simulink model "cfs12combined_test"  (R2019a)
settings: configuration reference "configurationSettings" (kept in a data dictionary, not in this file)
undefined symbols (not defined in the file or in its folder): algo_cfs1_fp, algo_cfs2_fp

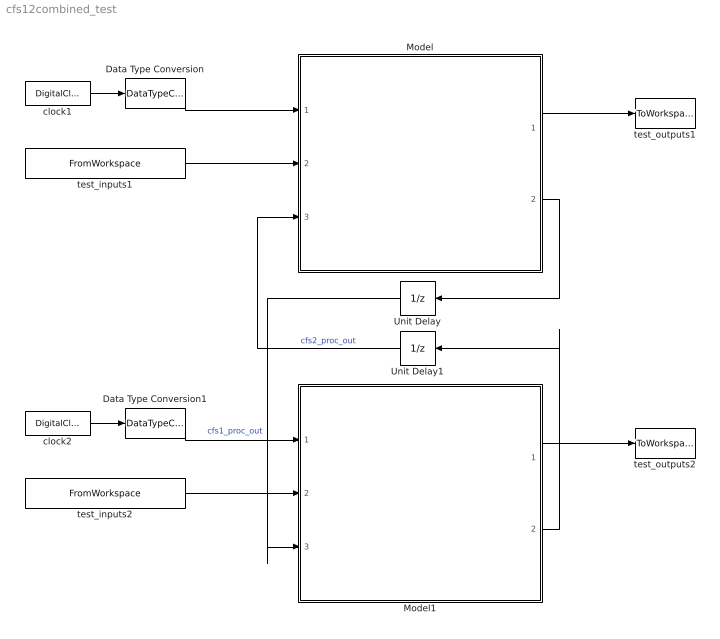
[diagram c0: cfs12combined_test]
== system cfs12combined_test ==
  Data Type Conversion : DataTypeConversion  OutDataTypeStr=single
  Data Type Conversion1 : DataTypeConversion  OutDataTypeStr=single
  Model : ModelReference  ModelNameDialog=algo_cfs1.slx  SimulationMode=Normal  ModelReferenceVersion=1.801  SimulationMode=Normal
  Model1 : ModelReference  ModelNameDialog=algo_cfs2.slx  SimulationMode=Normal  ModelReferenceVersion=1.795  SimulationMode=Normal
  Unit Delay : UnitDelay  SampleTime=-1  HasFrameUpgradeWarning=on
  Unit Delay1 : UnitDelay  SampleTime=-1  HasFrameUpgradeWarning=on
  clock1 : DigitalClock  SampleTime=algo_cfs1_fp.timing.dt
  clock2 : DigitalClock  SampleTime=algo_cfs1_fp.timing.dt
  test_inputs1 : FromWorkspace  VariableName=algo_cfs1_inbus1  OutDataTypeStr=Bus: algo_cfs1_inBus  SampleTime=algo_cfs1_fp.timing.dt  Interpolate=off  OutputAfterFinalValue=Holding final value
  test_inputs2 : FromWorkspace  VariableName=algo_cfs2_inbus1  OutDataTypeStr=Bus: algo_cfs2_inBus  SampleTime=algo_cfs2_fp.timing.dt  Interpolate=off  OutputAfterFinalValue=Holding final value
  test_outputs1 : ToWorkspace  VariableName=simout1  SaveFormat=Timeseries  SampleTime=-1
  test_outputs2 : ToWorkspace  VariableName=simout2  SaveFormat=Timeseries  SampleTime=-1
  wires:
  Model1/2 -> Unit Delay1/1
  clock2/1 -> Data Type Conversion1/1
  Unit Delay1/1 -> Model/3  "cfs2_proc_out"
  Model1/1 -> test_outputs2/1
  Data Type Conversion1/1 -> Model1/1
  Model/1 -> test_outputs1/1
  test_inputs2/1 -> Model1/2
  Data Type Conversion/1 -> Model/1
  Model/2 -> Unit Delay/1
  Unit Delay/1 -> Model1/3  "cfs1_proc_out"
  test_inputs1/1 -> Model/2
  clock1/1 -> Data Type Conversion/1
